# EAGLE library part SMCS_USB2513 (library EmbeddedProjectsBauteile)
USB 2.0 Hi-Speed Hub Controller
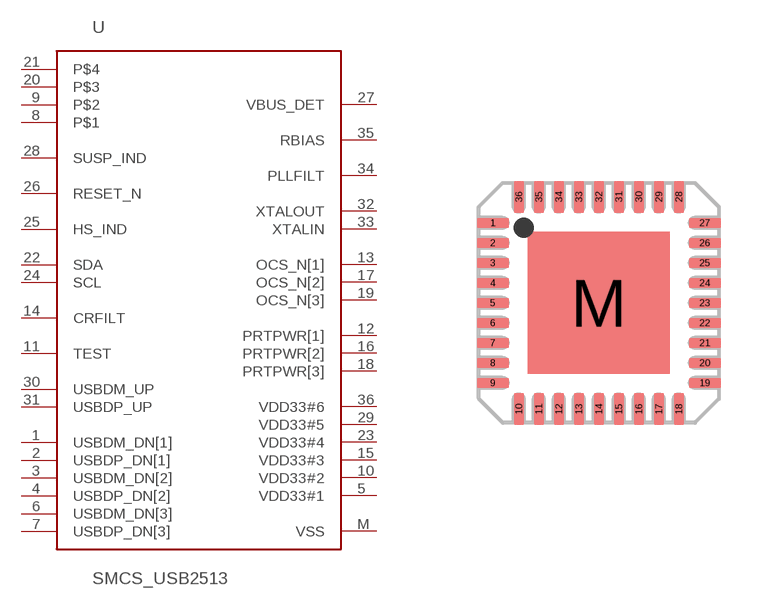
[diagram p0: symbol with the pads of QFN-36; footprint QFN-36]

Designator prefix -

## SMCS_USB2513  [QFN-36]
1  USBDM_DN[1]
2  USBDP_DN[1]
3  USBDM_DN[2]
4  USBDP_DN[2]
5  VDD33#1  sup
6  USBDM_DN[3]
7  USBDP_DN[3]
8  P$1  nc
9  P$2  nc
10  VDD33#2  sup
11  TEST
12  PRTPWR[1]
13  OCS_N[1]
14  CRFILT
15  VDD33#3  sup
16  PRTPWR[2]
17  OCS_N[2]
18  PRTPWR[3]
19  OCS_N[3]
20  P$3  nc
21  P$4  nc
22  SDA
23  VDD33#4  sup
24  SCL
25  HS_IND
26  RESET_N
27  VBUS_DET
28  SUSP_IND
29  VDD33#5  sup
30  USBDM_UP
31  USBDP_UP
32  XTALOUT
33  XTALIN
34  PLLFILT
35  RBIAS
36  VDD33#6  sup
M  VSS  pwr

## Footprint QFN-36 (pad centres in mm)
36-pin QFN
smd 0.8 x 0.25: 1 -2.65,2; 2 -2.65,1.5; 3 -2.65,1; 4 -2.65,0.5; 5 -2.65,0; 6 -2.65,-0.5; 7 -2.65,-1; 8 -2.65,-1.5; 9 -2.65,-2; 19 2.65,-2; 20 2.65,-1.5; 21 2.65,-1; 22 2.65,-0.5; 23 2.65,0; 24 2.65,0.5; 25 2.65,1; 26 2.65,1.5; 27 2.65,2
smd 0.25 x 0.8: 10 -2,-2.66; 11 -1.5,-2.66; 12 -1,-2.66; 13 -0.5,-2.66; 14 0,-2.66; 15 0.5,-2.66; 16 1,-2.66; 17 1.5,-2.66; 18 2,-2.66; 28 2,2.65; 29 1.5,2.65; 30 1,2.65; 31 0.5,2.65; 32 0,2.65; 33 -0.5,2.65; 34 -1,2.65; 35 -1.5,2.65; 36 -2,2.65
smd 3.55 x 3.55: M 0,0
